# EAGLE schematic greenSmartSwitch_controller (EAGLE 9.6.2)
DATABASE: Z:\Eigene Dateien\Anwendungsdaten\Eagle\partdb\exp.txt
Assembly variants: Std

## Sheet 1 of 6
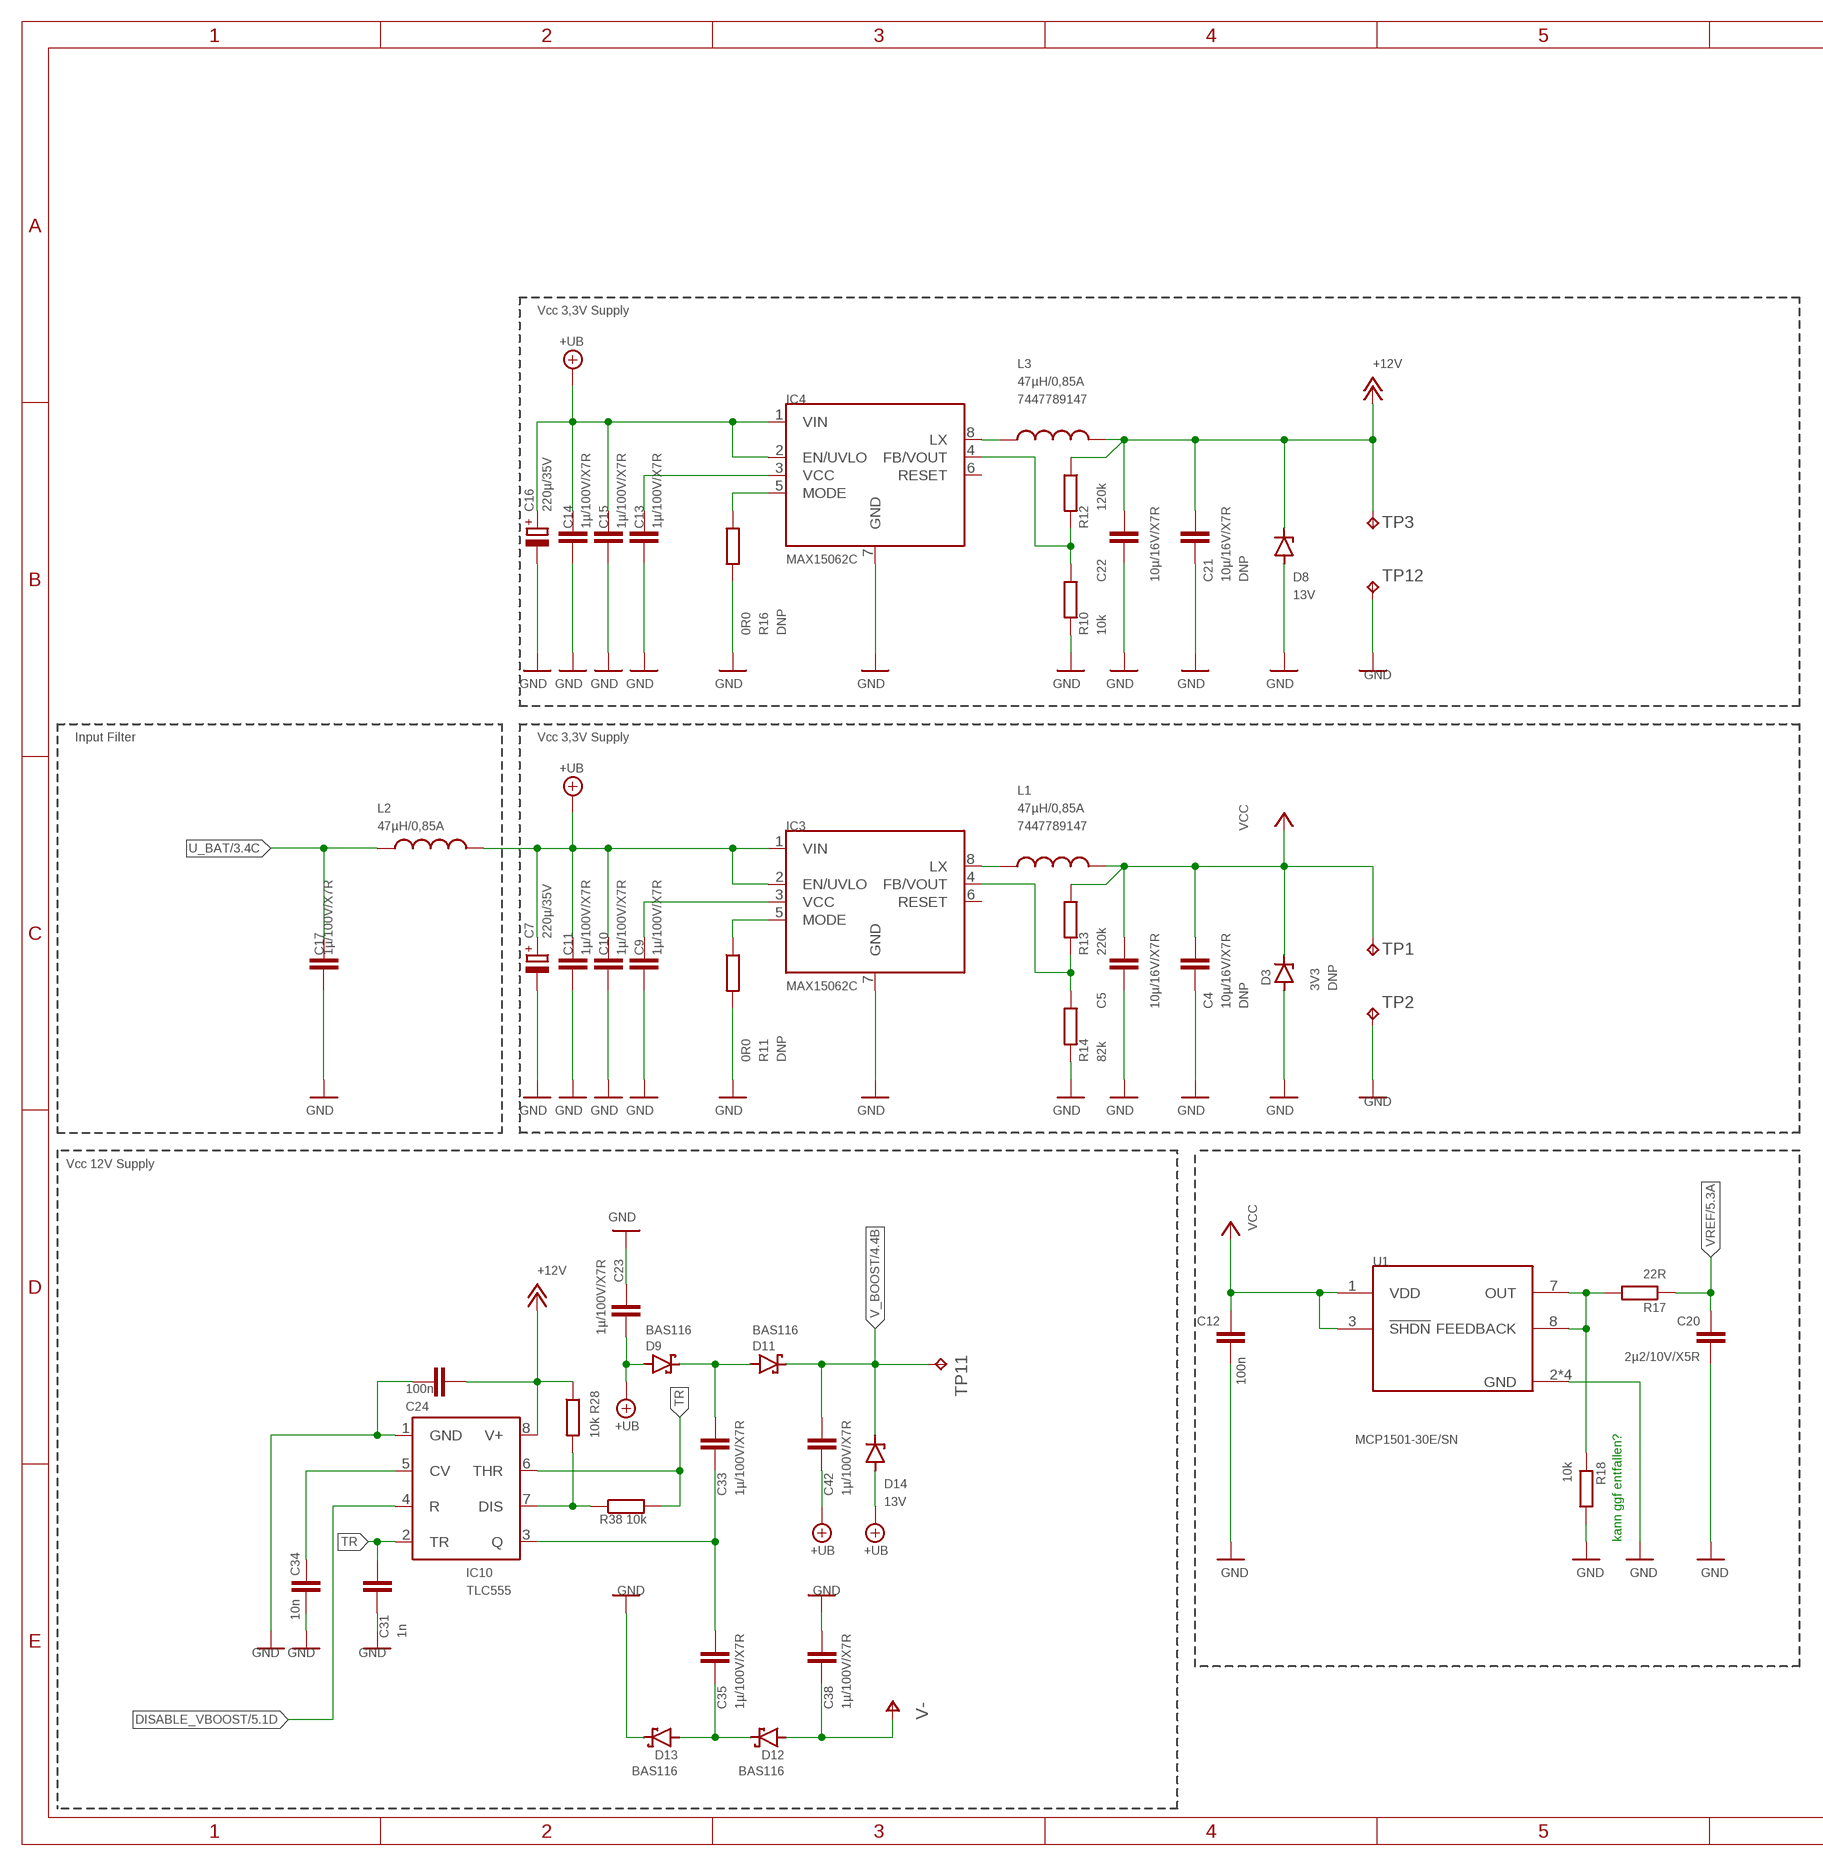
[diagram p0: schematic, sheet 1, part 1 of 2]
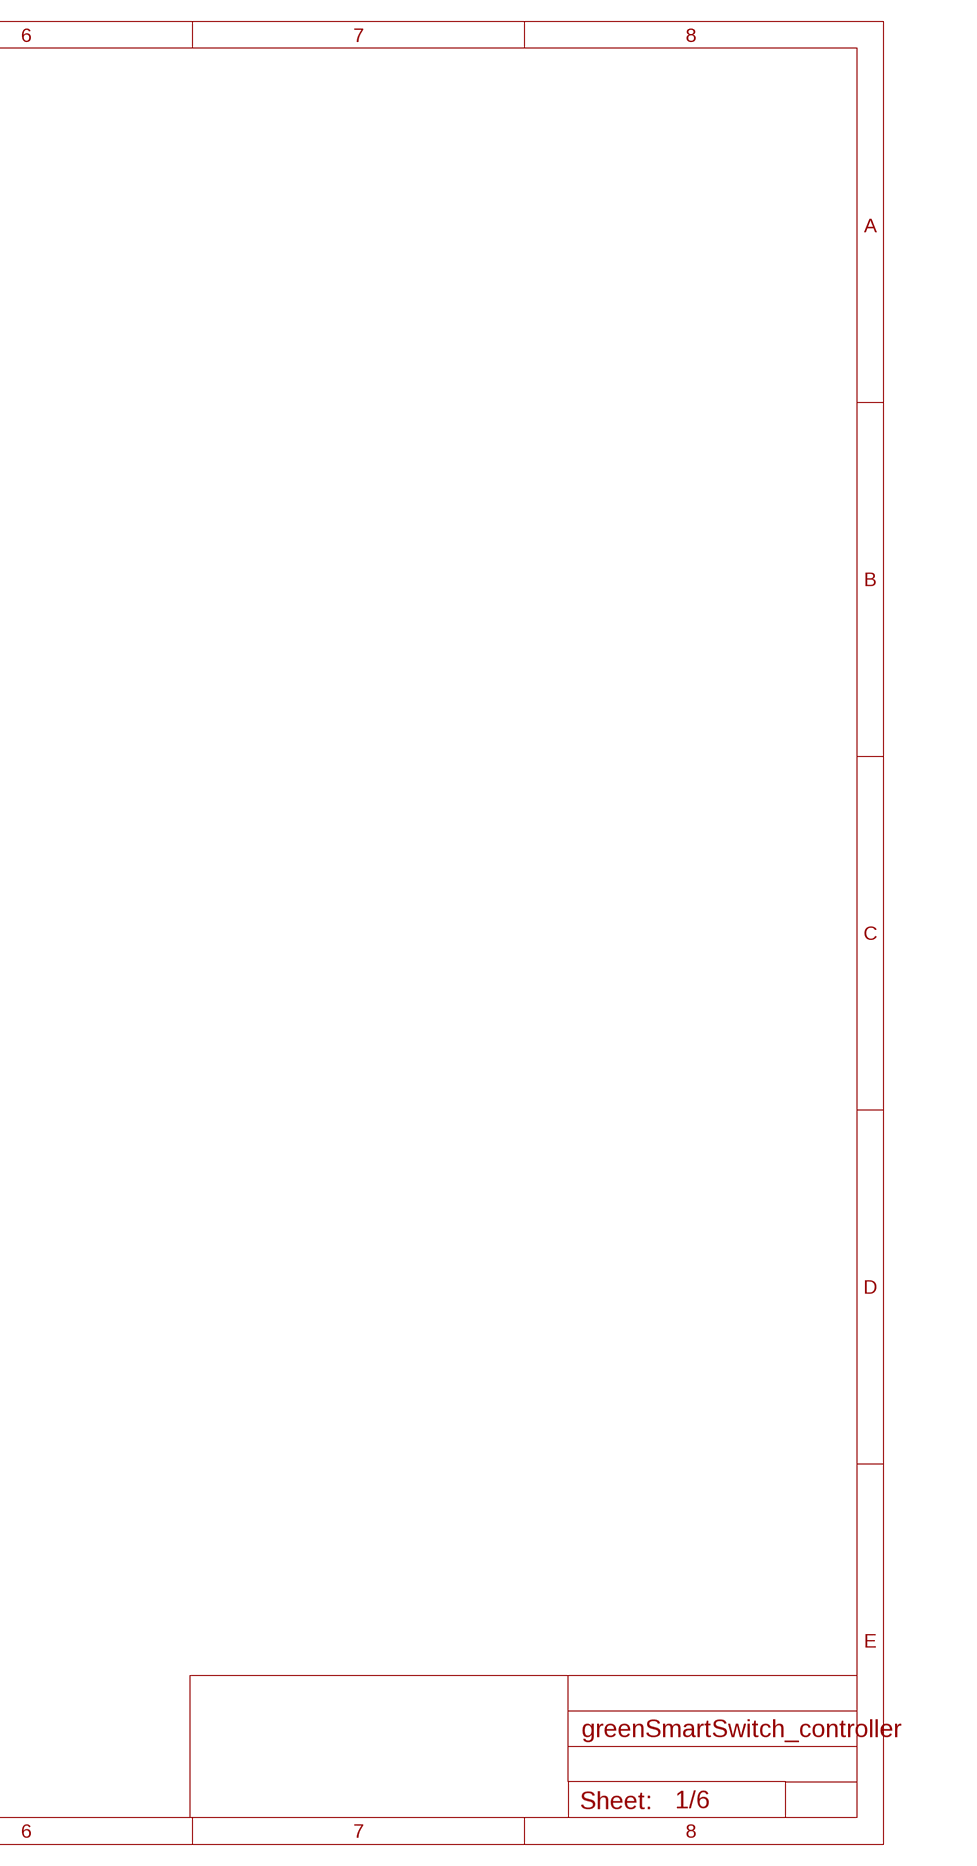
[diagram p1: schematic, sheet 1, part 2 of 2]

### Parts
C4  10µ/16V/X7R  C-EUC1210  [C1210]
C5  10µ/16V/X7R  C-EUC1210  [C1210]
C7  220µ/35V  CPOL-EUE3.5-8  [E3,5-8]
C9  1µ/100V/X7R  C-EUC1210  [C1210]
C10  1µ/100V/X7R  C-EUC1210  [C1210]
C11  1µ/100V/X7R  C-EUC1210  [C1210]
C12  100n  C-EUC0603  [C0603]
C13  1µ/100V/X7R  C-EUC1210  [C1210]
C14  1µ/100V/X7R  C-EUC1210  [C1210]
C15  1µ/100V/X7R  C-EUC1210  [C1210]
C16  220µ/35V  CPOL-EUE3.5-8  [E3,5-8]
C17  1µ/100V/X7R  C-EUC1210  [C1210]
C20  2µ2/10V/X5R  C-EUC0603  [C0603]
C21  10µ/16V/X7R  C-EUC1210  [C1210]
C22  10µ/16V/X7R  C-EUC1210  [C1210]
C23  1µ/100V/X7R  C-EUC1210  [C1210]
C24  100n  C-EUC0603  [C0603]
C31  1n  C-EUC0603  [C0603]
C33  1µ/100V/X7R  C-EUC1210  [C1210]
C34  10n  C-EUC0603  [C0603]
C35  1µ/100V/X7R  C-EUC1210  [C1210]
C38  1µ/100V/X7R  C-EUC1210  [C1210]
C42  1µ/100V/X7R  C-EUC1210  [C1210]
D3  3V3  ZENER-DIODESOD80C  [SOD80C]
D8  13V  ZENER-DIODESOD80C  [SOD80C]
D9  BAS116  BAS70  [SOT23]
D11  BAS116  BAS70  [SOT23]
D12  BAS116  BAS70  [SOT23]
D13  BAS116  BAS70  [SOT23]
D14  13V  ZENER-DIODESOD80C  [SOD80C]
IC3  MAX15062C  MAX15062A  [8TDFN]
IC4  MAX15062C  MAX15062A  [8TDFN]
IC10  TLC555  [SO8]
L1  47µH/0,85A  WE-PD_7332_PLASTIC_7447789147  [WE-PD_7332/7345_PLASTIC_BASE]
L2  47µH/0,85A  WE-PD_7332_PLASTIC_7447789147  [WE-PD_7332/7345_PLASTIC_BASE]
L3  47µH/0,85A  WE-PD_7332_PLASTIC_7447789147  [WE-PD_7332/7345_PLASTIC_BASE]
R10  10k  R-EU_R0603  [R0603]
R11  0R0  R-EU_R0603  [R0603]
R12  120k  R-EU_R0603  [R0603]
R13  220k  R-EU_R0603  [R0603]
R14  82k  R-EU_R0603  [R0603]
R16  0R0  R-EU_R0603  [R0603]
R17  22R  R-EU_R0603  [R0603]
R18  10k  R-EU_R0603  [R0603]
R28  10k  R-EU_R0603  [R0603]
R38  10k  R-EU_R0603  [R0603]
TP1  TP_0.6  [TP_0.6]
TP2  TP_0.6  [TP_0.6]
TP3  TP_0.6  [TP_0.6]
TP11  TP_0.6  [TP_0.6]
TP12  TP_0.6  [TP_0.6]
U1  MCP1501-30E/SN  MCP1501-40E/SN  [SOIC127P600X175-8N]

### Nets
+12V: C21.2 C22.2 C24.1 D8.C IC10.8(V+) L3.2 R12.1 R28.1 TP3.TP ; also sheet 2,4
+UB: C7.+ C10.2 C11.2 C14.2 C15.2 C16.+ C23.2 C42.1 D9.1(A) D14.A IC3.1(VIN) IC3.2(EN/UVLO) IC4.1(VIN) IC4.2(EN/UVLO) L2.2 ; also sheet 2
DISABLE_VBOOST: IC10.4(R) ; also sheet 5
GND: C4.1 C5.1 C7.- C9.1 C10.1 C11.1 C12.2 C13.1 C14.1 C15.1 C16.- C17.1 C20.2 C21.1 C22.1 C23.1 C24.2 C31.1 C34.1 C38.2 D3.A D8.A D13.3(C) IC3.7(GND) IC4.7(GND) IC10.1(GND) R10.2 R11.2 R14.2 R16.2 R18.2 TP2.TP TP12.TP U1.2(GND) U1.4(GND) U1.5(GND) U1.6(GND) ; also sheet 2,3,4,5,6
N$2: IC10.7(DIS) R28.2 R38.1
N$6: IC3.5(MODE) R11.1
N$8: C9.2 IC3.3(VCC)
N$21: IC3.4(FB/VOUT) R13.2 R14.1
N$23: C33.2 D9.3(C) D11.1(A)
N$26: C35.1 D12.3(C) D13.1(A)
N$36: C34.2 IC10.5(CV)
N$39: C33.1 C35.2 IC10.3(Q)
N$51: IC4.8(LX) L3.1
N$58: IC4.5(MODE) R16.1
N$60: C13.2 IC4.3(VCC)
N$61: IC4.4(FB/VOUT) R10.1 R12.2
N$91: IC3.8(LX) L1.1
N$119: R17.2 R18.1 U1.7(OUT) U1.8(FEEDBACK)
TR: C31.2 IC10.2(TR) IC10.6(THR) R38.2
U_BAT: C17.2 L2.1 ; also sheet 3
V-: C38.1 D12.1(A) ; also sheet 4
V_BOOST: C42.2 D11.3(C) D14.C TP11.TP ; also sheet 4
VCC: C4.2 C5.2 C12.1 D3.C L1.2 R13.1 TP1.TP U1.1(VDD) U1.3(!SHDN) ; also sheet 2,3,5,6
VREF: C20.1 R17.1 ; also sheet 5,6
Unconnected: IC3.6(RESET) IC4.6(RESET)

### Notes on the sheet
- Vcc 3,3V Supply
- 7447789147
- Input Filter | Vcc 3,3V Supply
- 7447789147
- Vcc 12V Supply
- kann ggf entfallen?

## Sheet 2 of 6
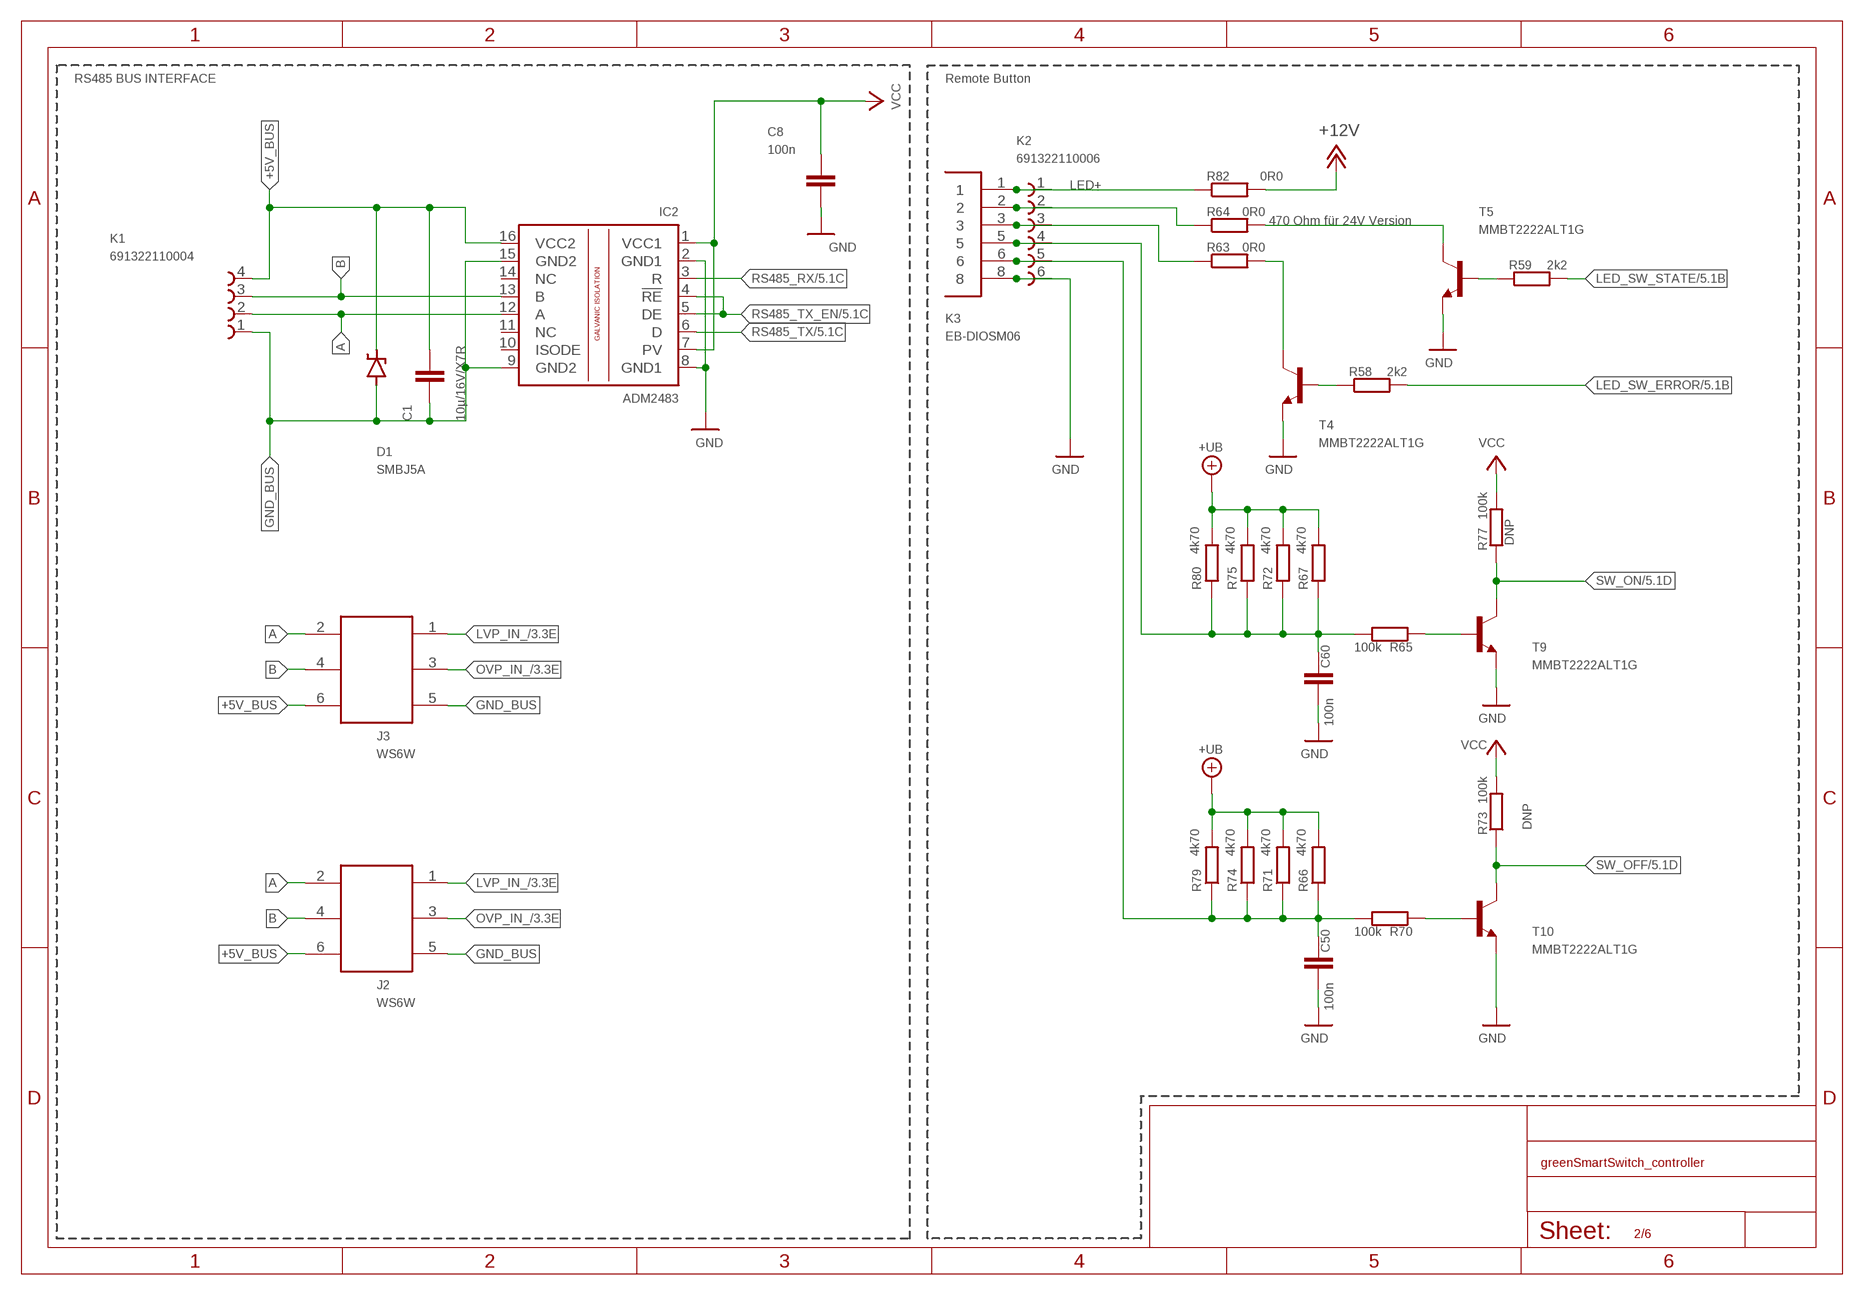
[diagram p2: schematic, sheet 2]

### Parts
C1  10µ/16V/X7R  C-EUC1210  [C1210]
C8  100n  C-EUC0603  [C0603]
C50  100n  C-EUC0603  [C0603]
C60  100n  C-EUC0603  [C0603]
D1  SMBJ5A  SUPPRESSOR-SMBJ  [SMBJ]
IC2  ADM2483  ISO1176  [SO-16DW]
J2  WS6W  61200621721  [61200621721]
J3  WS6W  61200621721  [61200621721]
K1  691322110004  [691322110004]
K2  691322110006  [691322110006]
K3  EB-DIOSM06  [PS/2-6]
R58  2k2  R-EU_R0603  [R0603]
R59  2k2  R-EU_R0603  [R0603]
R63  0R0  R-EU_R0603  [R0603]
R64  0R0  R-EU_R0603  [R0603]
R65  100k  R-EU_R0603  [R0603]
R66  4k70  R-EU_R1206  [R1206]
R67  4k70  R-EU_R1206  [R1206]
R70  100k  R-EU_R0603  [R0603]
R71  4k70  R-EU_R1206  [R1206]
R72  4k70  R-EU_R1206  [R1206]
R73  100k  R-EU_R0603  [R0603]
R74  4k70  R-EU_R1206  [R1206]
R75  4k70  R-EU_R1206  [R1206]
R77  100k  R-EU_R0603  [R0603]
R79  4k70  R-EU_R1206  [R1206]
R80  4k70  R-EU_R1206  [R1206]
R82  0R0  R-EU_R0603  [R0603]
T4  MMBT2222ALT1G  MMBT2222ALT1-NPN-SOT23-BEC  [SOT23-BEC]
T5  MMBT2222ALT1G  MMBT2222ALT1-NPN-SOT23-BEC  [SOT23-BEC]
T9  MMBT2222ALT1G  MMBT2222ALT1-NPN-SOT23-BEC  [SOT23-BEC]
T10  MMBT2222ALT1G  MMBT2222ALT1-NPN-SOT23-BEC  [SOT23-BEC]

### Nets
+5V_BUS: C1.2 D1.C IC2.16(VCC2) J2.6 J3.6 K1.4
+12V: R82.2 ; also sheet 1,4
+UB: R66.2 R67.2 R71.2 R72.2 R74.2 R75.2 R79.2 R80.2 ; also sheet 1
A: IC2.12(A) J2.2 J3.2 K1.2
B: IC2.13(B) J2.4 J3.4 K1.3
GND: C8.2 C50.2 C60.2 IC2.2(GND1) IC2.8(GND1) K2.6 K3.8 T4.E T5.E T9.E T10.E ; also sheet 1,3,4,5,6
GND_BUS: C1.1 D1.A IC2.9(GND2) IC2.15(GND2) J2.5 J3.5 K1.1
LED_SW_ERROR: R58.2 ; also sheet 5
LED_SW_STATE: R59.2 ; also sheet 5
LVP_IN_: J2.1 J3.1 ; also sheet 3
N$4: C60.1 K2.4 K3.5 R65.2 R67.1 R72.1 R75.1 R80.1
N$9: K2.1 K3.1 R82.1
N$14: C50.1 K2.5 K3.6 R66.1 R70.2 R71.1 R74.1 R79.1
N$15: R64.2 T5.C
N$17: K2.2 K3.2 R64.1
N$18: K2.3 K3.3 R63.1
N$25: R63.2 T4.C
N$27: R58.1 T4.B
N$30: R65.1 T9.B
N$32: R70.1 T10.B
N$33: R59.1 T5.B
OVP_IN_: J2.3 J3.3 ; also sheet 3
RS485_RX: IC2.3(R) ; also sheet 5
RS485_TX: IC2.6(D) ; also sheet 5
RS485_TX_EN: IC2.4(!RE) IC2.5(DE) ; also sheet 5
SW_OFF: R73.1 T10.C ; also sheet 5
SW_ON: R77.1 T9.C ; also sheet 5
VCC: C8.1 IC2.1(VCC1) IC2.7(PV) R73.2 R77.2 ; also sheet 1,3,5,6
Unconnected: IC2.10(ISODE) IC2.11(NC) IC2.14(NC)

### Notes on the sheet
- RS485 BUS INTERFACE | Remote Button
- LED+
- 470 Ohm für 24V Version

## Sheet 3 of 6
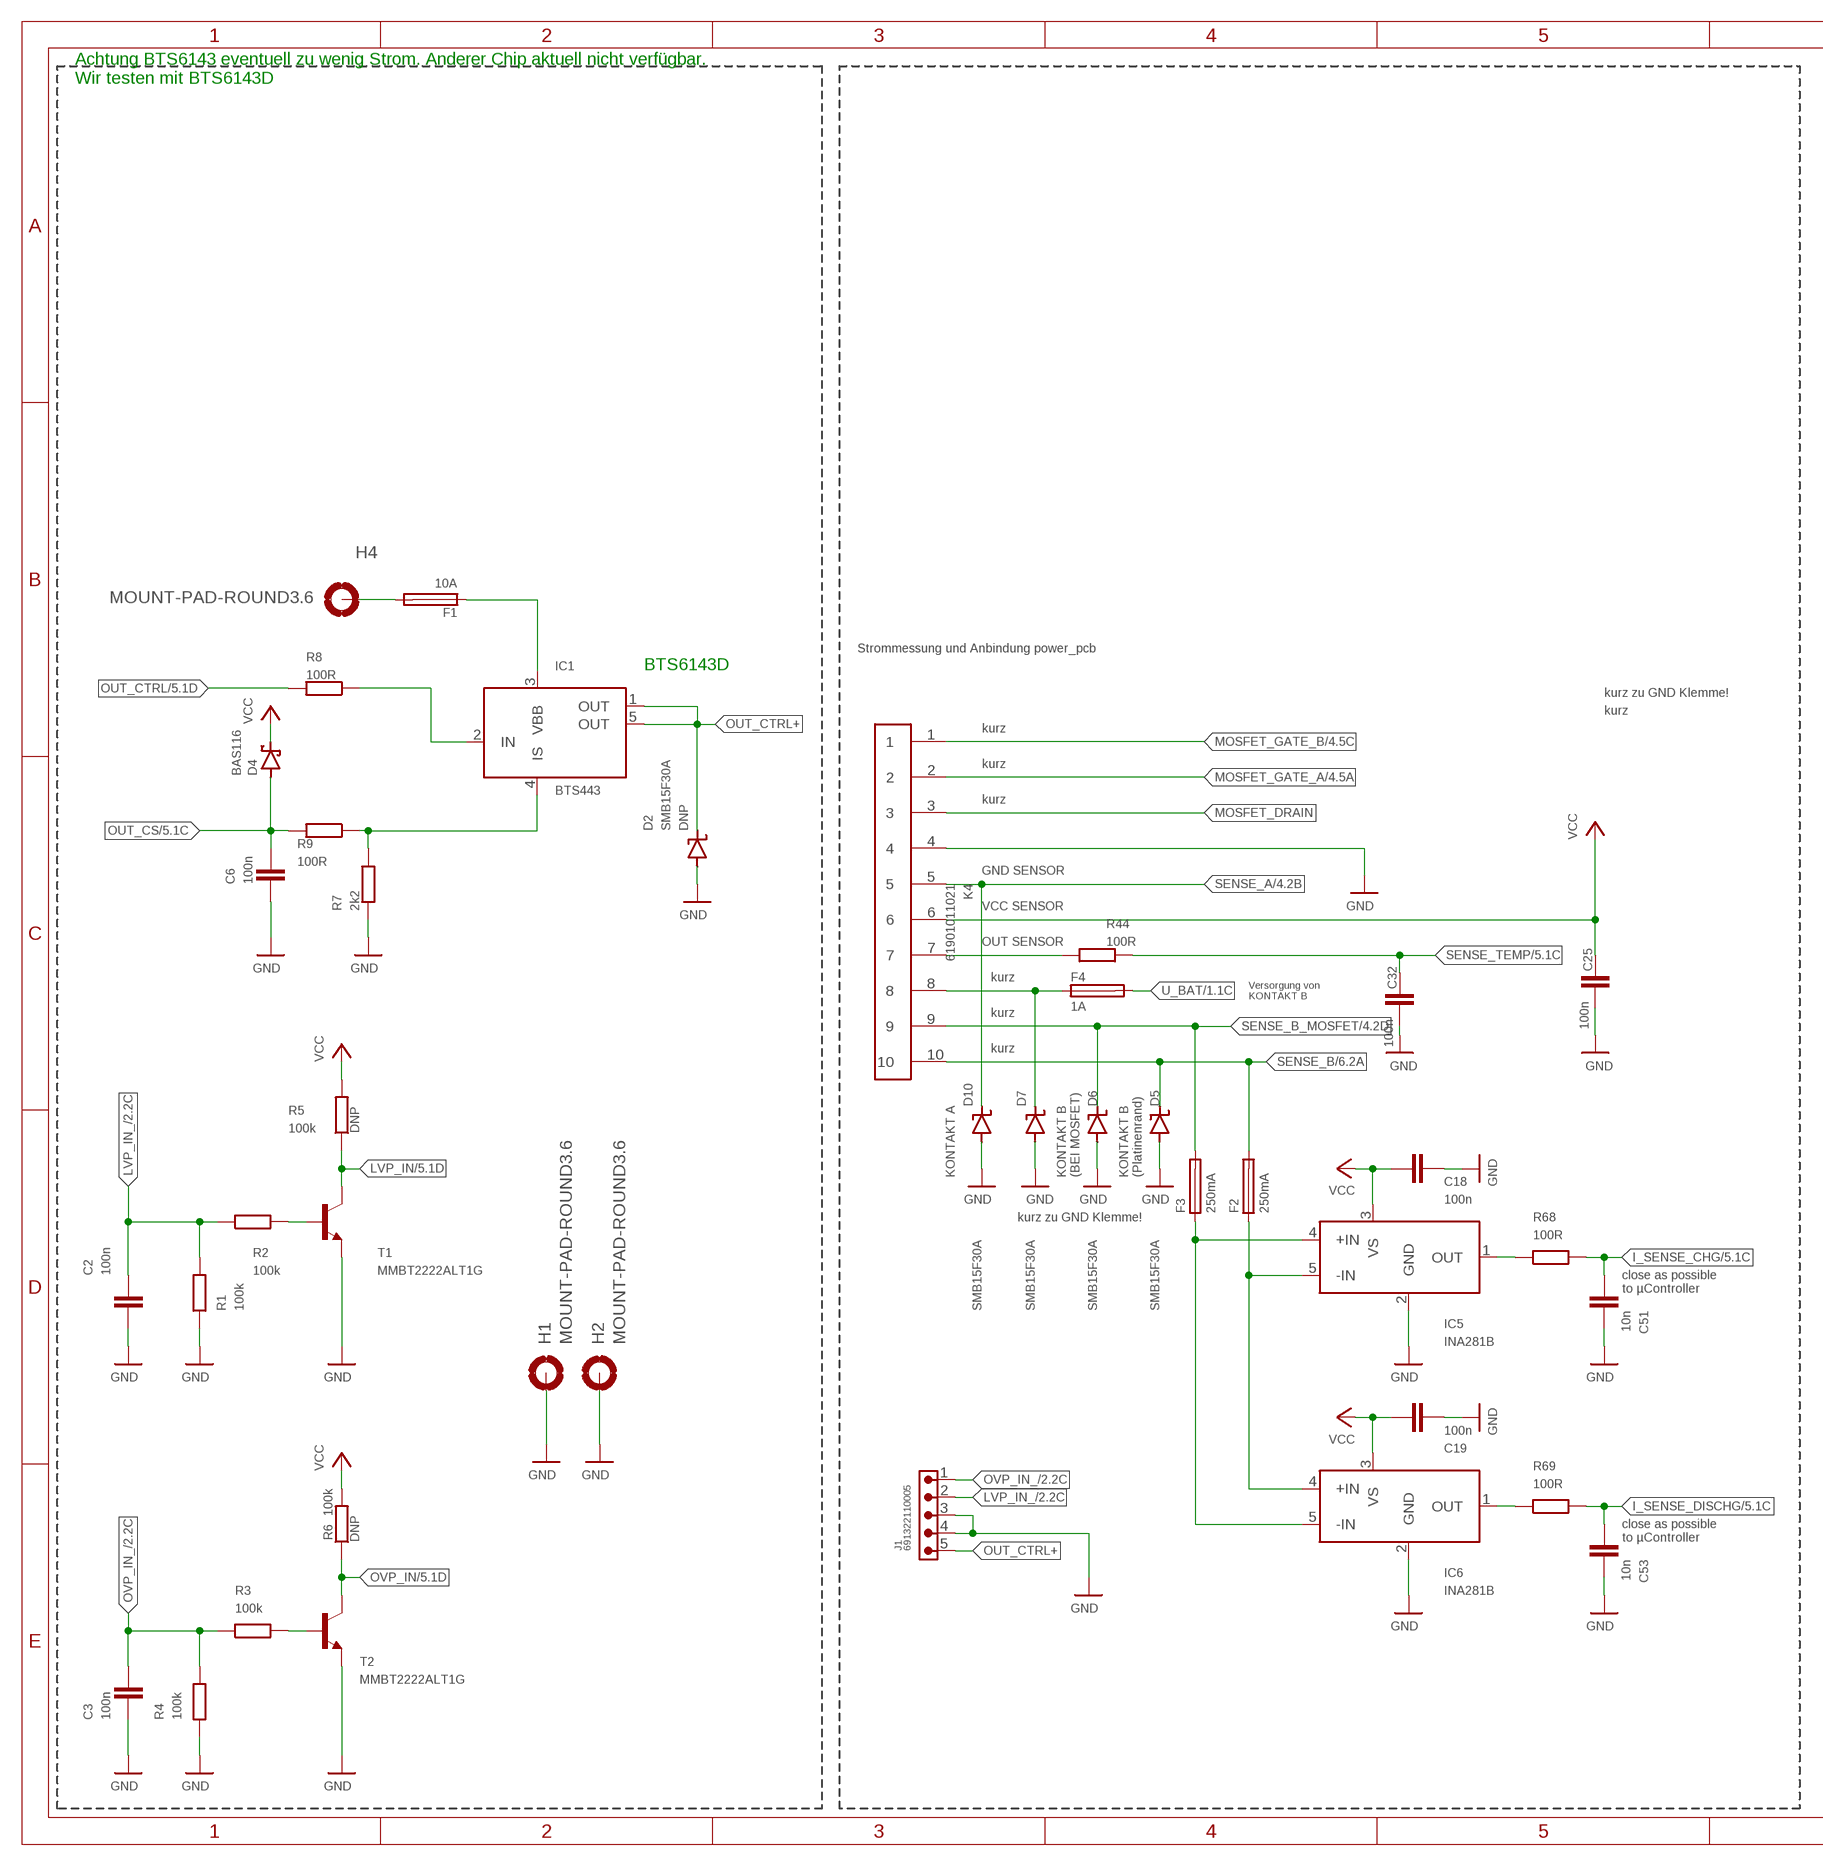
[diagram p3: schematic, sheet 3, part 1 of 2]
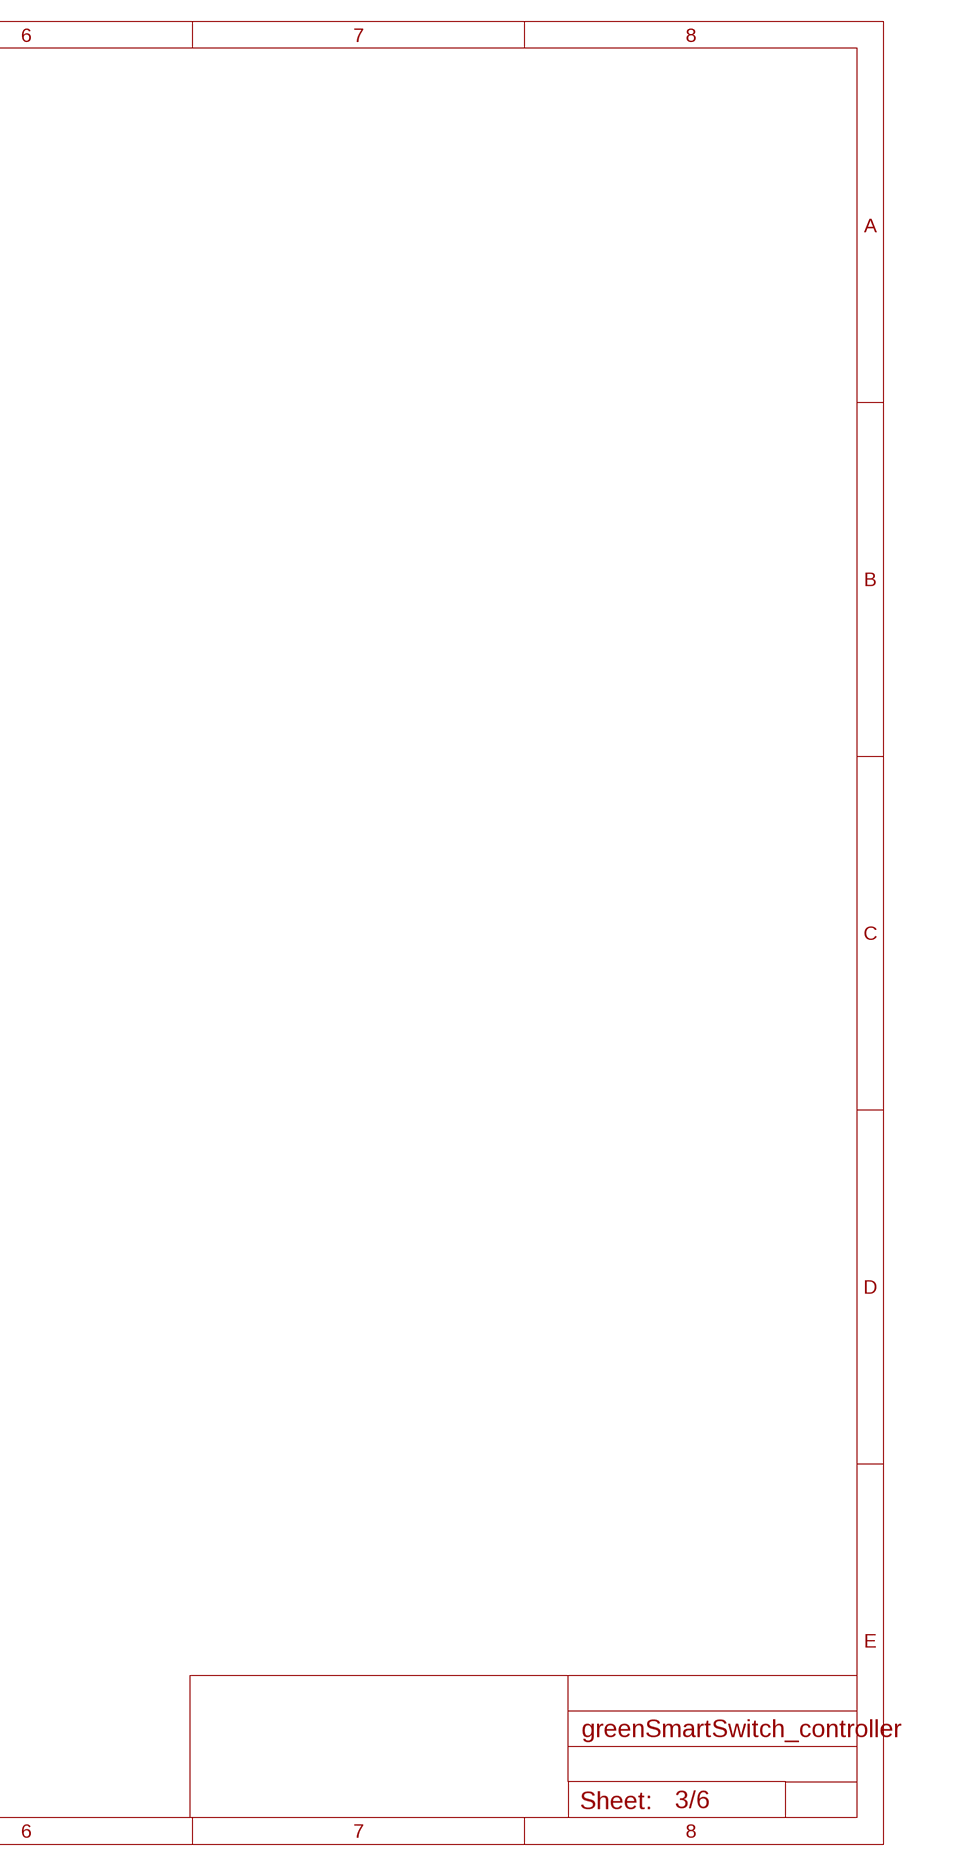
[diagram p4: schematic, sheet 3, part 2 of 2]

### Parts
C2  100n  C-EUC0603  [C0603]
C3  100n  C-EUC0603  [C0603]
C6  100n  C-EUC0603  [C0603]
C18  100n  C-EUC0603  [C0603]
C19  100n  C-EUC0603  [C0603]
C25  100n  C-EUC0603  [C0603]
C32  100n  C-EUC0603  [C0603]
C51  10n  C-EUC0603  [C0603]
C53  10n  C-EUC0603  [C0603]
D2  SMB15F30A  SUPPRESSOR-SMBJ  [SMBJ]
D4  BAS116  BAS70  [SOT23]
D5  SMB15F30A  SUPPRESSOR-SMBJ  [SMBJ]
D6  SMB15F30A  SUPPRESSOR-SMBJ  [SMBJ]
D7  SMB15F30A  SUPPRESSOR-SMBJ  [SMBJ]
D10  SMB15F30A  SUPPRESSOR-SMBJ  [SMBJ]
F1  10A  SSQ250-1K  [SSQ(2410)]
F2  250mA  SSQ250-1K  [SSQ(2410)]
F3  250mA  SSQ250-1K  [SSQ(2410)]
F4  1A  SSQ250-1K  [SSQ(2410)]
H1  MOUNT-PAD-ROUND3.6  [3,6-PAD]
H2  MOUNT-PAD-ROUND3.6  [3,6-PAD]
H4  MOUNT-PAD-ROUND3.6  [3,6-PAD]
IC1  BTS443  [PG-TO252-5-11]
IC5  INA281B  [SOT23-5]
IC6  INA281B  [SOT23-5]
J1  691322110005  [691322110005]
K4  61901011021  [61901011021]
R1  100k  R-EU_R0603  [R0603]
R2  100k  R-EU_R0603  [R0603]
R3  100k  R-EU_R0603  [R0603]
R4  100k  R-EU_R0603  [R0603]
R5  100k  R-EU_R0603  [R0603]
R6  100k  R-EU_R0603  [R0603]
R7  2k2  R-EU_R0603  [R0603]
R8  100R  R-EU_R0603  [R0603]
R9  100R  R-EU_R0603  [R0603]
R44  100R  R-EU_R0603  [R0603]
R68  100R  R-EU_R0603  [R0603]
R69  100R  R-EU_R0603  [R0603]
T1  MMBT2222ALT1G  MMBT2222ALT1-NPN-SOT23-BEC  [SOT23-BEC]
T2  MMBT2222ALT1G  MMBT2222ALT1-NPN-SOT23-BEC  [SOT23-BEC]

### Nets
GND: C2.1 C3.1 C6.1 C18.2 C19.2 C25.2 C32.2 C51.1 C53.1 D2.A D5.A D6.A D7.A D10.A H1.B3,6(MOUNT) H2.B3,6(MOUNT) IC5.2(GND) IC6.2(GND) J1.3 J1.4 K4.4 R1.1 R4.1 R7.2 T1.E T2.E ; also sheet 1,2,4,5,6
I_SENSE_CHG: C51.2 R68.2 ; also sheet 5
I_SENSE_DISCHG: C53.2 R69.2 ; also sheet 5
LVP_IN: R5.1 T1.C ; also sheet 5
LVP_IN_: C2.2 J1.2 R1.2 R2.1 ; also sheet 2
MOSFET_DRAIN: K4.3
MOSFET_GATE_A: K4.2 ; also sheet 4
MOSFET_GATE_B: K4.1 ; also sheet 4
N$1: K4.7 R44.2
N$10: IC6.1(OUT) R69.1
N$13: F3.1 IC5.4(+IN) IC6.5(-IN)
N$20: F1.2 H4.B3,6(MOUNT)
N$24: F2.1 IC5.5(-IN) IC6.4(+IN)
N$35: R2.2 T1.B
N$37: IC5.1(OUT) R68.1
N$40: R3.2 T2.B
N$47: D7.C F4.1 K4.8
N$68: IC1.4(IS) R7.1 R9.1
N$70: IC1.2(IN) R8.1
N$71: F1.1 IC1.3(VBB)
OUT_CS: C6.2 D4.1(A) R9.2 ; also sheet 5
OUT_CTRL: R8.2 ; also sheet 5
OUT_CTRL+: D2.C IC1.1(OUT) IC1.5(OUT) J1.5
OVP_IN: R6.1 T2.C ; also sheet 5
OVP_IN_: C3.2 J1.1 R3.1 R4.2 ; also sheet 2
SENSE_A: D10.C K4.5 ; also sheet 4,6
SENSE_B: D5.C F2.2 K4.10 ; also sheet 6
SENSE_B_MOSFET: D6.C F3.2 K4.9 ; also sheet 4
SENSE_TEMP: C32.1 R44.1 ; also sheet 5
U_BAT: F4.2 ; also sheet 1
VCC: C18.1 C19.1 C25.1 D4.3(C) IC5.3(VS) IC6.3(VS) K4.6 R5.2 R6.2 ; also sheet 1,2,5,6

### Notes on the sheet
- Achtung BTS6143 eventuell zu wenig Strom. Anderer Chip aktuell nicht verfügbar. 
  Wir testen mit BTS6143D
- Strommessung und Anbindung power_pcb
- BTS6143D
- kurz zu GND Klemme!
- kurz
- kurz
- kurz
- kurz
- GND SENSOR
- VCC SENSOR
- OUT SENSOR
- kurz
- Versorgung von
  KONTAKT B
- kurz
- kurz
- KONTAKT A
- KONTAKT B
  (BEI MOSFET)
- KONTAKT B 
  (Platinenrand)
- kurz zu GND Klemme!
- close as possible
  to µController
- close as possible
  to µController

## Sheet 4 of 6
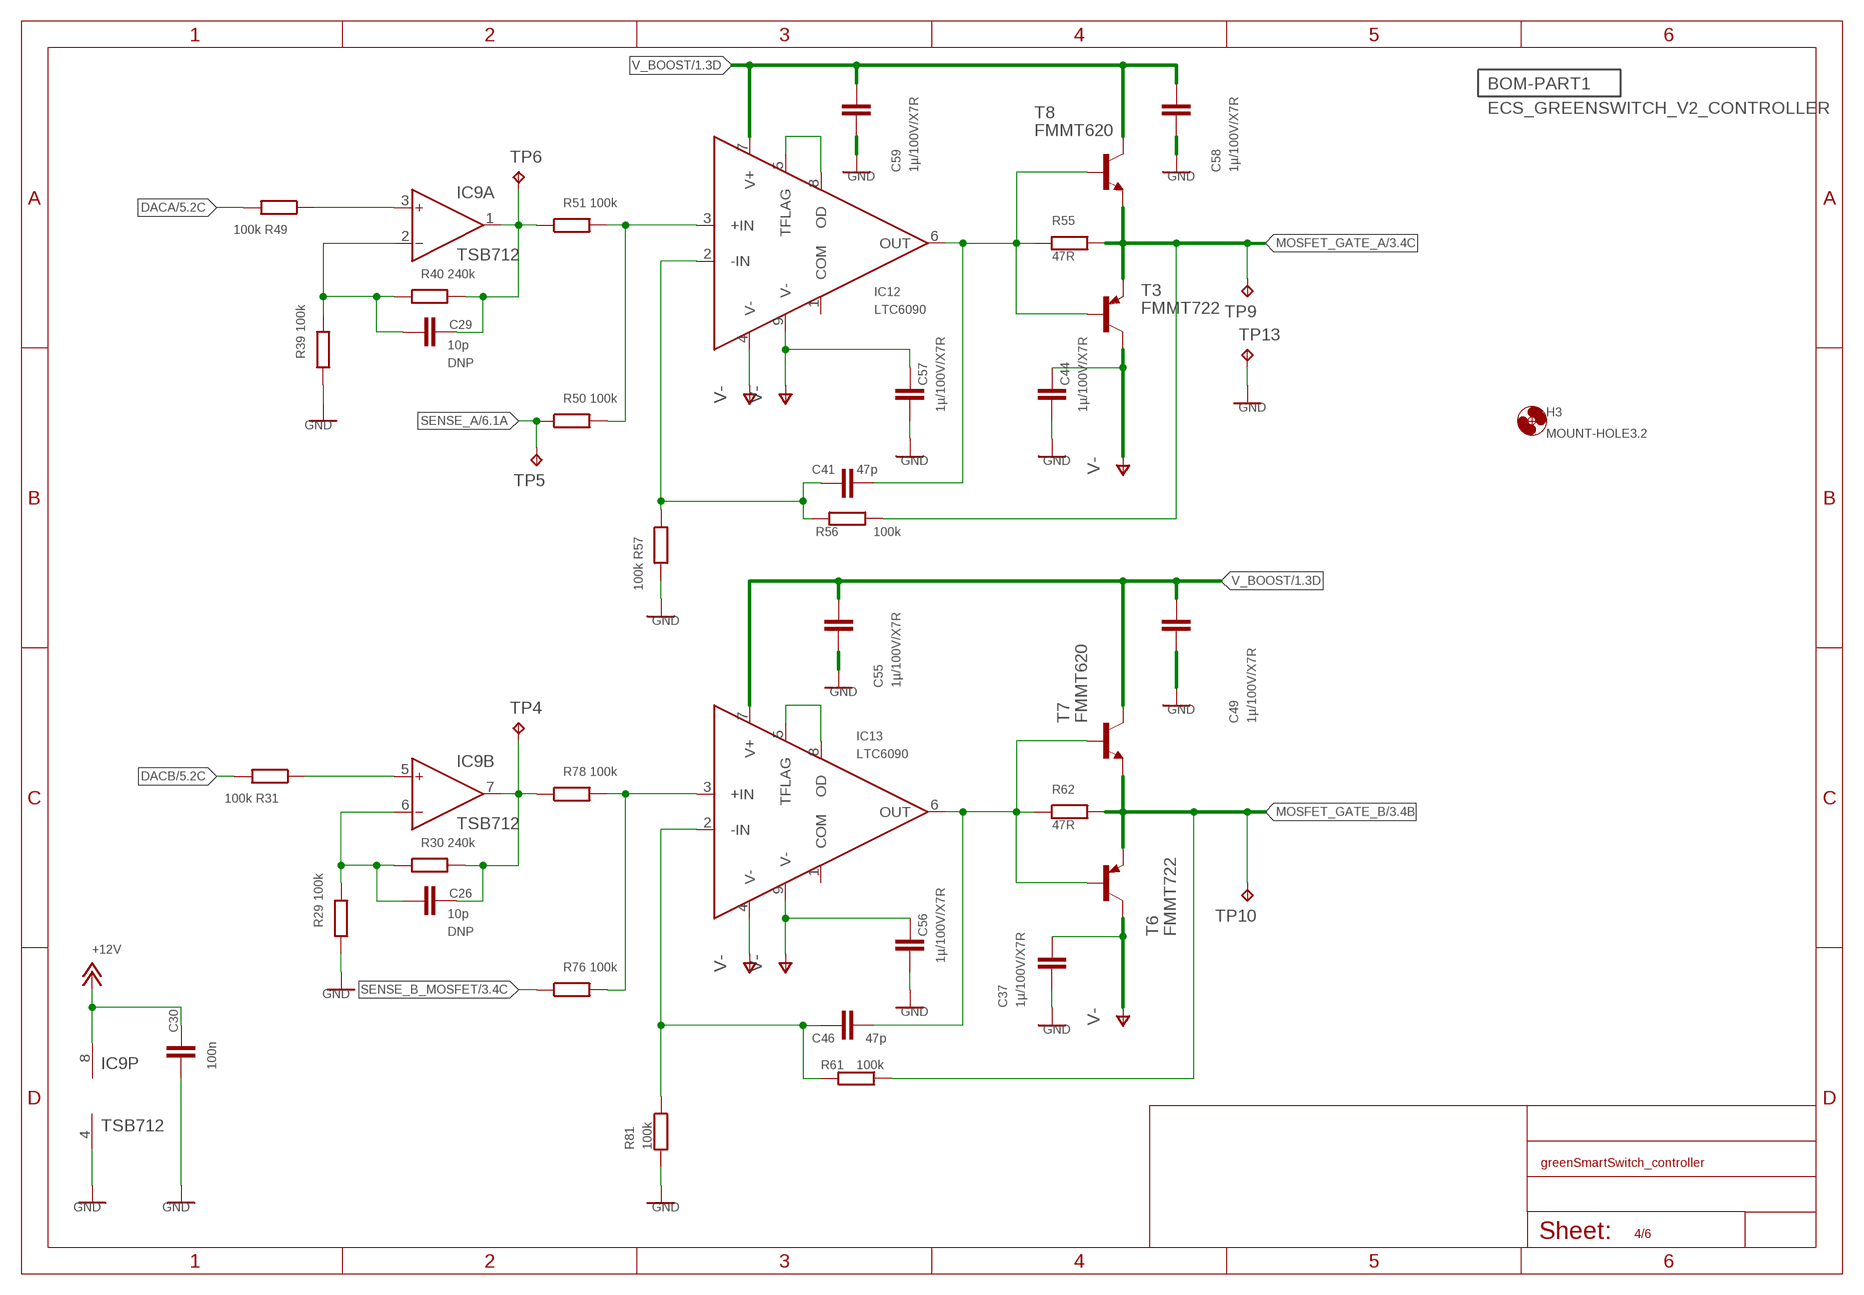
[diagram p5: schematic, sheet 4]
BOM-PART1 (BOM-PART): BOM: INCLUDE; PARTNO: PT066; QTY: 1

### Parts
C26  10p  C-EUC0603  [C0603]
C29  10p  C-EUC0603  [C0603]
C30  100n  C-EUC0603  [C0603]
C37  1µ/100V/X7R  C-EUC1210  [C1210]
C41  47p  C-EUC0603  [C0603]
C44  1µ/100V/X7R  C-EUC1210  [C1210]
C46  47p  C-EUC0603  [C0603]
C49  1µ/100V/X7R  C-EUC1210  [C1210]
C55  1µ/100V/X7R  C-EUC1210  [C1210]
C56  1µ/100V/X7R  C-EUC1210  [C1210]
C57  1µ/100V/X7R  C-EUC1210  [C1210]
C58  1µ/100V/X7R  C-EUC1210  [C1210]
C59  1µ/100V/X7R  C-EUC1210  [C1210]
H3  MOUNT-HOLE3.2  [3,2]
IC9  TSB712  TS912  [SO8]
IC12  LTC6090  [S8E(SOIC)]
IC13  LTC6090  [S8E(SOIC)]
R29  100k  R-EU_R0603  [R0603]
R30  240k  R-EU_R0603  [R0603]
R31  100k  R-EU_R0603  [R0603]
R39  100k  R-EU_R0603  [R0603]
R40  240k  R-EU_R0603  [R0603]
R49  100k  R-EU_R0603  [R0603]
R50  100k  R-EU_R0603  [R0603]
R51  100k  R-EU_R0603  [R0603]
R55  47R  R-EU_R0603  [R0603]
R56  100k  R-EU_R0603  [R0603]
R57  100k  R-EU_R0603  [R0603]
R61  100k  R-EU_R0603  [R0603]
R62  47R  R-EU_R0603  [R0603]
R76  100k  R-EU_R0603  [R0603]
R78  100k  R-EU_R0603  [R0603]
R81  100k  R-EU_R0603  [R0603]
T3  FMMT722  BC857A-PNP-SOT23-BEC  [SOT23-BEC]
T6  FMMT722  BC857A-PNP-SOT23-BEC  [SOT23-BEC]
T7  FMMT620  BC847  [SOT23]
T8  FMMT620  BC847  [SOT23]
TP4  TP_0.6  [TP_0.6]
TP5  TP_0.6  [TP_0.6]
TP6  TP_0.6  [TP_0.6]
TP9  TP_0.6  [TP_0.6]
TP10  TP_0.6  [TP_0.6]
TP13  TP_0.6  [TP_0.6]

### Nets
+12V: C30.1 IC9.8(P:V+) ; also sheet 1,2
DACA: R49.2 ; also sheet 5
DACA_: IC9.3(A:IN+) R49.1
DACB: R31.2 ; also sheet 5
DACB_: IC9.5(B:IN+) R31.1
GND: C30.2 C37.2 C44.2 C49.2 C55.2 C56.2 C57.2 C58.2 C59.2 IC9.4(P:V-) R29.1 R39.1 R57.2 R81.2 TP13.TP ; also sheet 1,2,3,5,6
MOSFET_GATE_A: R55.2 R56.1 T3.E T8.2(E) TP9.TP ; also sheet 3
MOSFET_GATE_B: R61.1 R62.2 T6.E T7.2(E) TP10.TP ; also sheet 3
N$19: C46.2 IC13.2(-IN) R61.2 R81.1
N$22: C41.2 IC12.2(-IN) R56.2 R57.1
N$29: C29.1 IC9.1(A:OUT) R40.2 R51.1 TP6.TP
N$38: IC12.5(TFLAG) IC12.8(OD)
N$43: C26.2 IC9.6(B:IN-) R29.2 R30.1
N$46: IC13.5(TFLAG) IC13.8(OD)
N$54: IC12.3(+IN) R50.2 R51.2
N$56: C26.1 IC9.7(B:OUT) R30.2 R78.1 TP4.TP
N$59: IC13.3(+IN) R76.2 R78.2
N$66: C29.2 IC9.2(A:IN-) R39.2 R40.1
PREDRIVER_A: C41.1 IC12.6(OUT) R55.1 T3.B T8.1(B)
PREDRIVER_B: C46.1 IC13.6(OUT) R62.1 T6.B T7.1(B)
SENSE_A: R50.1 TP5.TP ; also sheet 3,6
SENSE_B_MOSFET: R76.1 ; also sheet 3
V-: C37.1 C44.1 C56.1 C57.1 IC12.4(V-) IC12.9(V-) IC13.4(V-) IC13.9(V-) T3.C T6.C ; also sheet 1
V_BOOST: C49.1 C55.1 C58.1 C59.1 IC12.7(V+) IC13.7(V+) T7.3(C) T8.3(C) ; also sheet 1
Unconnected: IC12.1(COM) IC13.1(COM)

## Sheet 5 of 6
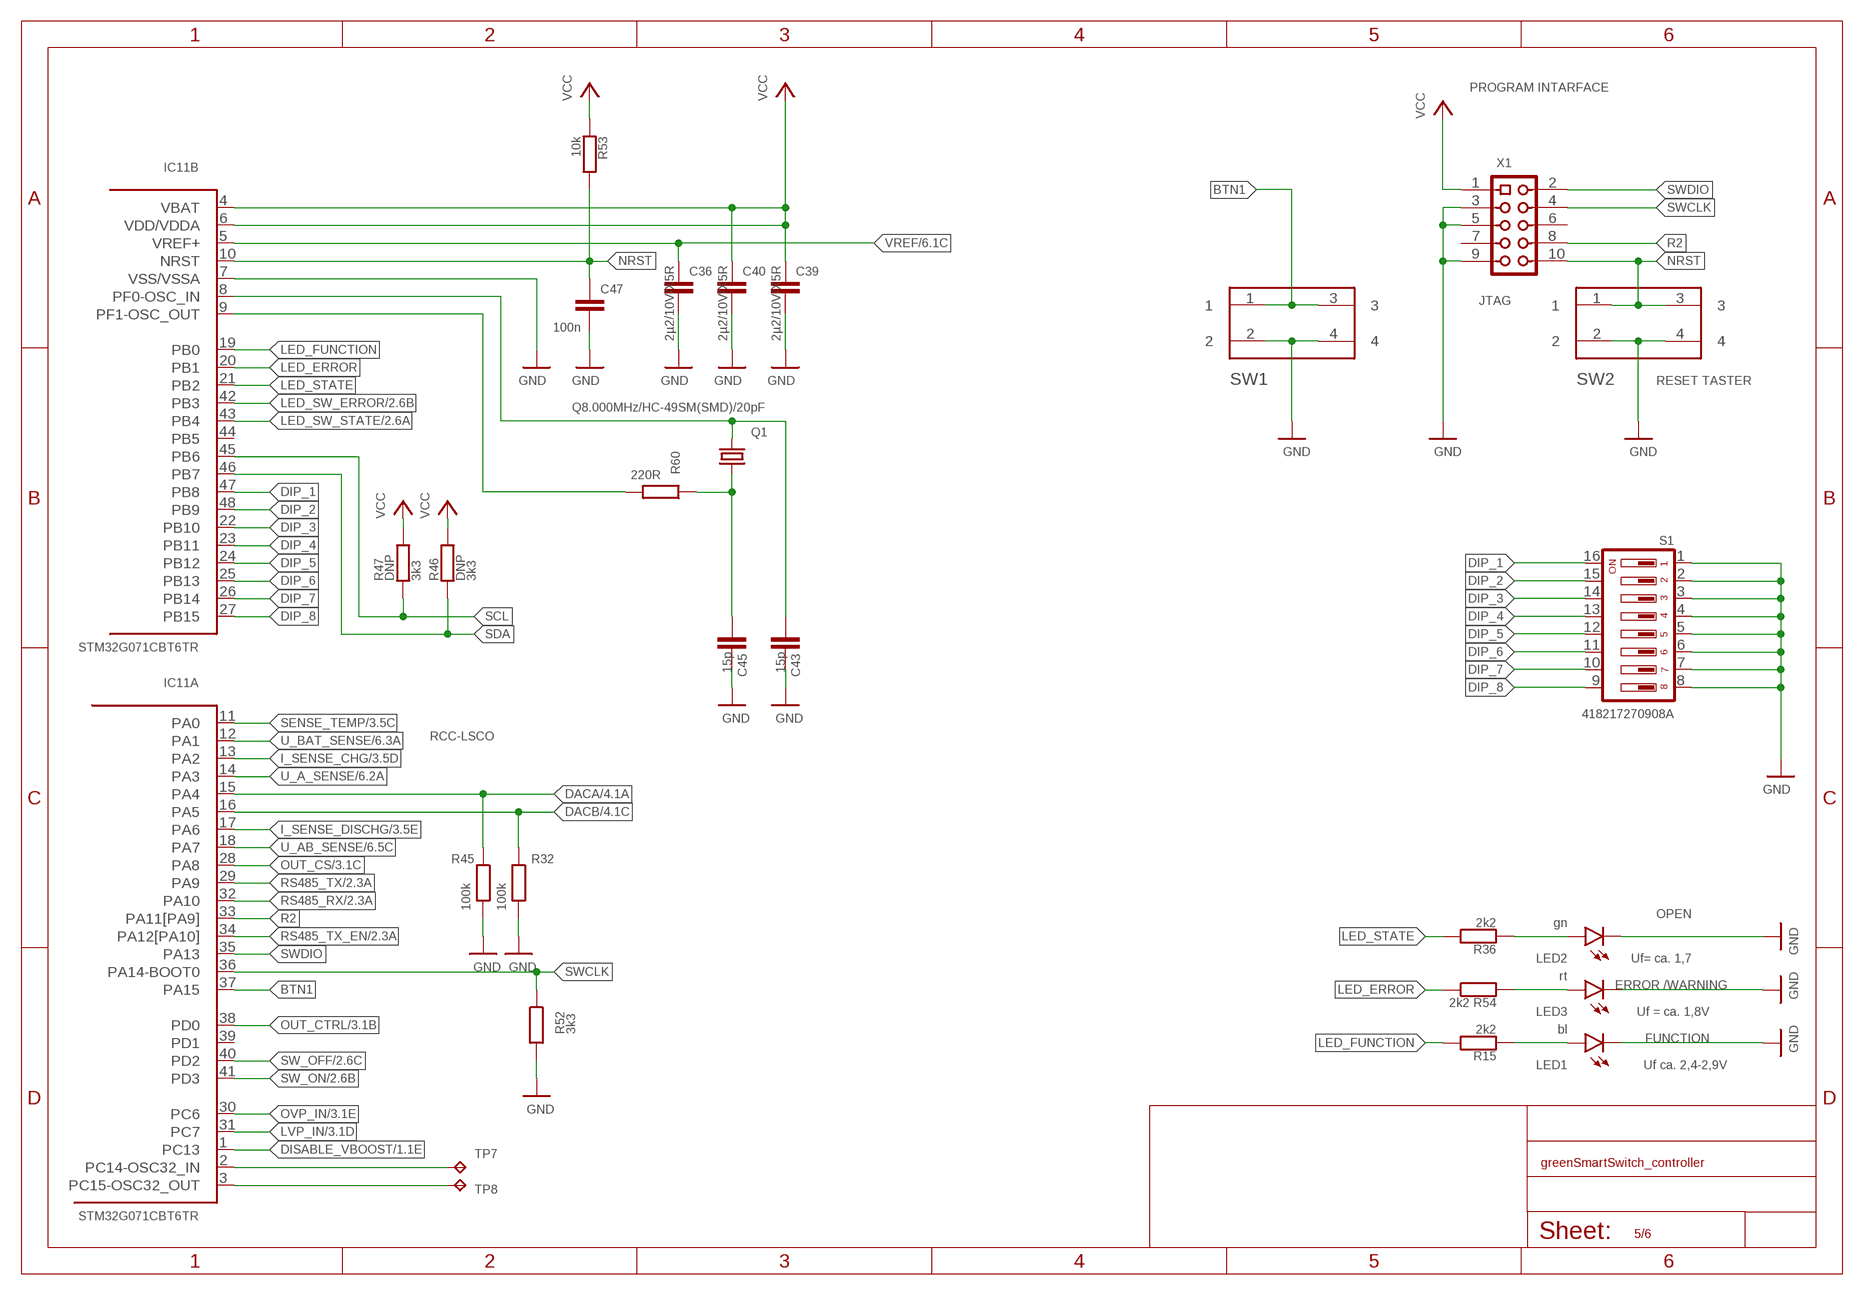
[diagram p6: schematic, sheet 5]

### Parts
C36  2µ2/10V/X5R  C-EUC0603  [C0603]
C39  2µ2/10V/X5R  C-EUC0603  [C0603]
C40  2µ2/10V/X5R  C-EUC0603  [C0603]
C43  15p  C-EUC0603  [C0603]
C45  15p  C-EUC0603  [C0603]
C47  100n  C-EUC0603  [C0603]
IC11  STM32G071CBT6TR  STM32G070CB  [LQFP48]
LED1  bl  LEDCHIPLED_0603  [CHIPLED_0603]
LED2  gn  LEDCHIPLED_0603  [CHIPLED_0603]
LED3  rt  LEDCHIPLED_0603  [CHIPLED_0603]
Q1  Q8.000MHz/HC-49SM(SMD)/20pF  CRYSTALHC49UP  [HC49UP]
R15  2k2  R-EU_R0603  [R0603]
R32  100k  R-EU_R0603  [R0603]
R36  2k2  R-EU_R0603  [R0603]
R45  100k  R-EU_R0603  [R0603]
R46  3k3  R-EU_R0603  [R0603]
R47  3k3  R-EU_R0603  [R0603]
R52  3k3  R-EU_R0603  [R0603]
R53  10k  R-EU_R0603  [R0603]
R54  2k2  R-EU_R0603  [R0603]
R60  220R  R-EU_R0603  [R0603]
S1  418217270908A  DA08  [DA-08]
SW1  430182095816  [430182095816]
SW2  430182095816  [430182095816]
TP7  TP_0.6  [TP_0.6]
TP8  TP_0.6  [TP_0.6]
X1  JTAG  PF2X5SMD1.27MM  [PF2X5SMD50MIL]

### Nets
BTN1: IC11.37(A:PA15) SW1.1 SW1.3
DACA: IC11.15(A:PA4) R45.1 ; also sheet 4
DACB: IC11.16(A:PA5) R32.1 ; also sheet 4
DIP_1: IC11.47(B:PB8) S1.16
DIP_2: IC11.48(B:PB9) S1.15
DIP_3: IC11.22(B:PB10) S1.14
DIP_4: IC11.23(B:PB11) S1.13
DIP_5: IC11.24(B:PB12) S1.12
DIP_6: IC11.25(B:PB13) S1.11
DIP_7: IC11.26(B:PB14) S1.10
DIP_8: IC11.27(B:PB15) S1.9
DISABLE_VBOOST: IC11.1(A:PC13) ; also sheet 1
GND: C36.2 C39.2 C40.2 C43.1 C45.1 C47.2 IC11.7(B:VSS/VSSA) LED1.C LED2.C LED3.C R32.2 R45.2 R52.2 S1.1 S1.2 S1.3 S1.4 S1.5 S1.6 S1.7 S1.8 SW1.2 SW1.4 SW2.2 SW2.4 X1.3 X1.5 X1.9 ; also sheet 1,2,3,4,6
I_SENSE_CHG: IC11.13(A:PA2) ; also sheet 3
I_SENSE_DISCHG: IC11.17(A:PA6) ; also sheet 3
LED_ERROR: IC11.20(B:PB1) R54.1
LED_FUNCTION: IC11.19(B:PB0) R15.1
LED_STATE: IC11.21(B:PB2) R36.1
LED_SW_ERROR: IC11.42(B:PB3) ; also sheet 2
LED_SW_STATE: IC11.43(B:PB4) ; also sheet 2
LVP_IN: IC11.31(A:PC7) ; also sheet 3
N$5: C43.2 IC11.8(B:PF0-OSC_IN) Q1.2
N$7: C45.2 Q1.1 R60.1
N$11: IC11.9(B:PF1-OSC_OUT) R60.2
N$12: LED2.A R36.2
N$16: IC11.2(A:PC14-OSC32_IN) TP7.TP
N$31: LED1.A R15.2
N$34: LED3.A R54.2
N$42: IC11.3(A:PC15-OSC32_OUT) TP8.TP
NRST: C47.1 IC11.10(B:NRST) R53.1 SW2.1 SW2.3 X1.10
OUT_CS: IC11.28(A:PA8) ; also sheet 3
OUT_CTRL: IC11.38(A:PD0) ; also sheet 3
OVP_IN: IC11.30(A:PC6) ; also sheet 3
R2: IC11.33(A:PA11[PA9]) X1.8
RS485_RX: IC11.32(A:PA10) ; also sheet 2
RS485_TX: IC11.29(A:PA9) ; also sheet 2
RS485_TX_EN: IC11.34(A:PA12[PA10]) ; also sheet 2
SCL: IC11.45(B:PB6) R47.1
SDA: IC11.46(B:PB7) R46.1
SENSE_TEMP: IC11.11(A:PA0) ; also sheet 3
SW_OFF: IC11.40(A:PD2) ; also sheet 2
SW_ON: IC11.41(A:PD3) ; also sheet 2
SWCLK: IC11.36(A:PA14-BOOT0) R52.1 X1.4
SWDIO: IC11.35(A:PA13) X1.2
U_A_SENSE: IC11.14(A:PA3) ; also sheet 6
U_AB_SENSE: IC11.18(A:PA7) ; also sheet 6
U_BAT_SENSE: IC11.12(A:PA1) ; also sheet 6
VCC: C39.1 C40.1 IC11.4(B:VBAT) IC11.6(B:VDD/VDDA) R46.2 R47.2 R53.2 X1.1 ; also sheet 1,2,3,6
VREF: C36.1 IC11.5(B:VREF+) ; also sheet 1,6
Unconnected: IC11.39(A:PD1) IC11.44(B:PB5) X1.6 X1.7

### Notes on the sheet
- PROGRAM INTARFACE
- RESET TASTER
- RCC-LSCO
- OPEN
- Uf= ca. 1,7
- ERROR /WARNING
- Uf = ca. 1,8V
- FUNCTION
- Uf ca. 2,4-2,9V

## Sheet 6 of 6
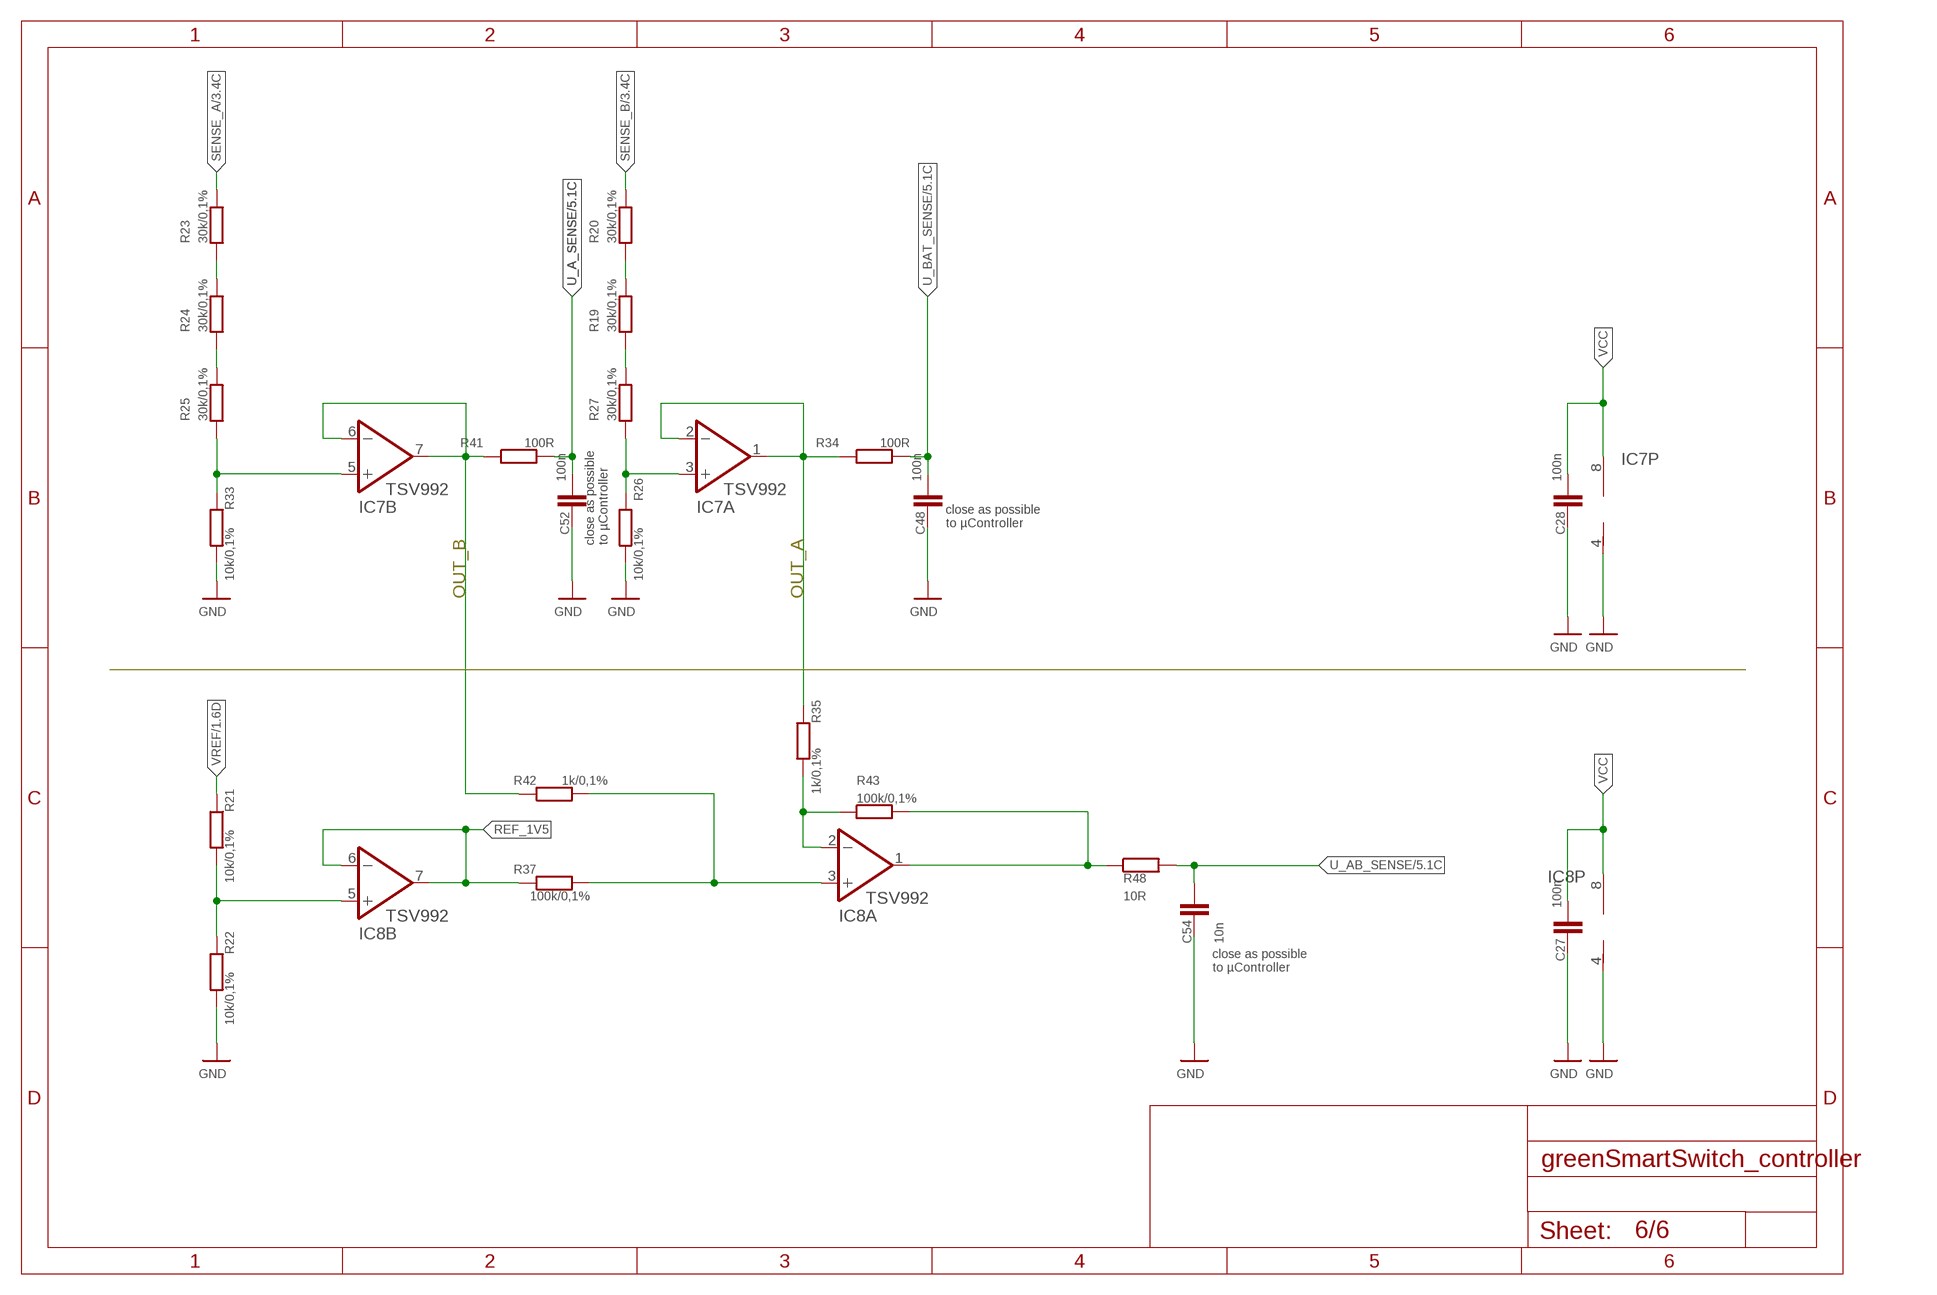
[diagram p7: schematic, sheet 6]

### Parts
C27  100n  C-EUC0603  [C0603]
C28  100n  C-EUC0603  [C0603]
C48  100n  C-EUC0603  [C0603]
C52  100n  C-EUC0603  [C0603]
C54  10n  C-EUC0603  [C0603]
IC7  TSV992  LT6231IS8  [S8]
IC8  TSV992  LT6231IS8  [S8]
R19  30k/0,1%  R-EU_R0603  [R0603]
R20  30k/0,1%  R-EU_R0603  [R0603]
R21  10k/0,1%  R-EU_R0603  [R0603]
R22  10k/0,1%  R-EU_R0603  [R0603]
R23  30k/0,1%  R-EU_R0603  [R0603]
R24  30k/0,1%  R-EU_R0603  [R0603]
R25  30k/0,1%  R-EU_R0603  [R0603]
R26  10k/0,1%  R-EU_R0603  [R0603]
R27  30k/0,1%  R-EU_R0603  [R0603]
R33  10k/0,1%  R-EU_R0603  [R0603]
R34  100R  R-EU_R0603  [R0603]
R35  1k/0,1%  R-EU_R0603  [R0603]
R37  100k/0,1%  R-EU_R0603  [R0603]
R41  100R  R-EU_R0603  [R0603]
R42  1k/0,1%  R-EU_R0603  [R0603]
R43  100k/0,1%  R-EU_R0603  [R0603]
R48  10R  R-EU_R0603  [R0603]

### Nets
GND: C27.1 C28.1 C48.1 C52.1 C54.1 IC7.4(P:V-) IC8.4(P:V-) R22.2 R26.2 R33.2 ; also sheet 1,2,3,4,5
N$3: R24.1 R25.2
N$28: IC7.1(A:OUT) IC7.2(A:-IN) R34.1 R35.1
N$41: IC7.6(B:-IN) IC7.7(B:OUT) R41.1 R42.1
N$44: IC8.2(A:-IN) R35.2 R43.1
N$45: IC8.3(A:+IN) R37.2 R42.2
N$48: IC7.3(A:+IN) R26.1 R27.1
N$49: R23.1 R24.2
N$50: R19.1 R27.2
N$52: R19.2 R20.1
N$55: IC8.5(B:+IN) R21.2 R22.1
N$57: IC7.5(B:+IN) R25.1 R33.1
N$9999: IC8.1(A:OUT) R43.2 R48.1
REF_1V5: IC8.6(B:-IN) IC8.7(B:OUT) R37.1
SENSE_A: R23.2 ; also sheet 3,4
SENSE_B: R20.2 ; also sheet 3
U_A_SENSE: C52.2 R41.2 ; also sheet 5
U_AB_SENSE: C54.2 R48.2 ; also sheet 5
U_BAT_SENSE: C48.2 R34.2 ; also sheet 5
VCC: C27.2 C28.2 IC7.8(P:V+) IC8.8(P:V+) ; also sheet 1,2,3,5
VREF: R21.1 ; also sheet 1,5

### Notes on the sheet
- close as possible
  to µController
- close as possible
  to µController
- OUT_B | OUT_A
- close as possible
  to µController

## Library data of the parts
C1 C5 C22 = rcl:C-EU: CAPACITOR, European symbol; PARTNO: C218; SPICEPREFIX: C
C2 C3 C6 C8 C25 C27 C28 C32 C48 C50 C52 C60 = resistor:C-EU: CAPACITOR, European symbol; PARTNO: C067
C4 C21 = rcl:C-EU: CAPACITOR, European symbol; DNP: T; PARTNO: C218; SPICEPREFIX: C
C7 C16 = rcl:CPOL-EU: POLARIZED CAPACITOR, European symbol; PARTNO: C194; SPICEPREFIX: C
C9-C11 C13-C15 C17 C23 C33 C35 C37 C38 C42 C44 C49 C55-C59 = rcl:C-EU: CAPACITOR, European symbol; PARTNO: C216; SPICEPREFIX: C
C12 C18 C19 C24 C30 C47 = rcl:C-EU: CAPACITOR, European symbol; PARTNO: C067; SPICEPREFIX: C
C20 C36 C39 C40 = rcl:C-EU: CAPACITOR, European symbol; PARTNO: C083; SPICEPREFIX: C
C26 C29 = rcl:C-EU: CAPACITOR, European symbol; DNP: T; PARTNO: C020; SPICEPREFIX: C
C31 = rcl:C-EU: CAPACITOR, European symbol; PARTNO: C043; SPICEPREFIX: C
C34 C51 C53 = rcl:C-EU: CAPACITOR, European symbol; PARTNO: C055; SPICEPREFIX: C
C41 C46 = rcl:C-EU: CAPACITOR, European symbol; PARTNO: C028; SPICEPREFIX: C
C43 C45 = resistor:C-EU: CAPACITOR, European symbol; PARTNO: C022
C54 = resistor:C-EU: CAPACITOR, European symbol; PARTNO: C055
D1 = diode:SUPPRESSOR-: Suppressor diode; PARTNO: D087
D2 = diode:SUPPRESSOR-: Suppressor diode; DNP: T; PARTNO: D211
D3 = diode:ZENER-DIODE: Z-Diode; DNP: T; PARTNO: D007
D4 D9 D11-D13 = diode:BAS70: Silicon Schottky Diodes; PARTNO: D204
D5-D7 D10 = diode:SUPPRESSOR-: Suppressor diode; PARTNO: D211
D8 D14 = diode:ZENER-DIODE: Z-Diode; PARTNO: D022
F1 = SSQ250-1K:SSQ250-1K: Square Ceramic Surface Mount Quick Acting Fuse; PARTNO: EM144
F2 F3 = SSQ250-1K:SSQ250-1K: Square Ceramic Surface Mount Quick Acting Fuse; PARTNO: EM186
F4 = SSQ250-1K:SSQ250-1K: Square Ceramic Surface Mount Quick Acting Fuse; PARTNO: EM216
H1 H2 H4 = holes:MOUNT-PAD-ROUND: MOUNTING PAD, round; BOM: EXCLUDE
H3 = holes:MOUNT-HOLE: MOUNTING HOLE with drill center marker; BOM: EXCLUDE; PARTNO: *
IC1 = BTS443:BTS443: Smart Highside Power Switch; PARTNO: IC367
IC2 = texas:ISO1176: ISOLATED RS-485 PROFIBUS TRANSCEIVER Source: Data sheet; MPN: ISO1176DW; OC_FARNELL: 1755037; OC_NEWARK: 13N4111; PARTNO: IC002
IC3 IC4 = MAX15062A:MAX15062A: 60V, 300mA, Ultra-Small, High-Efficiency, Synchronous Step-Down DC-DC Converters; PARTNO: IC292
IC5 IC6 = INA281B:INA281B: INA281-Q1 AEC-Q100, –4-V to 110-V, 1.3-MHz Current-Sense Amplifier; PARTNO: IC350
IC7 IC8 = linear-technology:LT6231: 215MHz, Rail-to-Rail Output, 1.1nV/Hz, 3.5mA Op Amp Source: http://cds.linear.com/docs/Datasheet/623012fb.pdf; MPN: LT6231IS8; OC_FARNELL: unknown; OC_NEWARK: 57M9356; PARTNO: IC222
IC9 = TS912:TS912: Rail-to-rail CMOS dual operational amplifier; PARTNO: IC347
IC10 = TLC555:TLC555: TLC555 LinCMOS™ Timer; PARTNO: IC322
IC11 = STM32G070CB:STM32G070CB: Arm® Cortex®-M0+ 32-bit MCU, 128 KB Flash, 36 KB RAM, 4x USART, timers, ADC, comm. I/Fs, 2.0-3.6V; PARTNO: IC321
IC12 IC13 = LTC6090:LTC6090: 140V CMOS Rail-to-Rail Output, Picoamp Input Current Op Amp; PARTNO: IC330
J1 = Wurth_Connectors_WR-TBL Pluggable Connector:691322110005: WR-TBL Serie 3221 - 3.50 mm Horizontal PCB Header KIND PROPERTIES Pitch 3.5 mm MATERIAL PROPERTIES Insulator Material PA66 Insulator Flammability Rating UL94 V-0 Contact Material Brass Contact Plating Tin GENERAL INFORMATION Operating Temperature -40 up to +105 °C Compliance RoHS ELECTRICAL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; DATASHEET-URL: https://www.we-online.com/catalog/datasheet/691322110005.pdf; IR-UL: 10A; IR-VDE: 10.5A; MOUNT: THT; PART-NUMBER: 691322110005; PARTNO: CON215; PINS: 5; PITCH: 3.5mm; TYPE: Horizontal; VALUE: 691322110005; WORKING-VOLTAGE-UL: 300V (AC); WORKING-VOLTAGE-VDE: 300V (AC)
J2 J3 = Wire-to-Board (rev18a):61200621721: WR-BHD 2.54mm Male Angled Box Header, 6 Pins=>Code : Con_WTB_BHD_2.54_Male_THT_WS_61200621721 Details see: http://katalog.we-online.de/en/em/612_0xx_217_21 Created 2014-06-05, Karrer Zheng 2014 (C) Würth Elektronik; PARTNO: CON398
K1 = Wuerth_Elektronik_eiCan_14_Terminal_Blocks_WR-TBL_2_0:691322110004: WR-TBL Serie 3221 - 3.50mm Horizontal PCB Header, 4 Pins; PARTNO: CON214
K2 = Wuerth_Elektronik_eiCan_14_Terminal_Blocks_WR-TBL_2_0:691322110006: WR-TBL Serie 3221 - 3.50mm Horizontal PCB Header, 6 Pins; PARTNO: CON413
K3 = EB-DIOS M06:EB-DIOSM06: EB-DIOS M06 6-pol. Mini-DIN-Buchse, vollgeschirmt; PARTNO: CON442
K4 = Wuerth_Elektronik_eiCan_09_Wire_to_Board_Connectors (1):61901011021: WR-WTB 2.54mm Right Angled Locking Header Bottom Locking, 10 Pins; PARTNO: CON058
L1-L3 = PowerMagnetics (rev18e):WE-PD_7332_PLASTIC: SMD Shielded Power Inductor; PARTNO: L110; WE-NUMBER: 7447789147/47uH
LED1 = led:LED: LED; PARTNO: D077
LED2 = led:LED: LED; PARTNO: D078
LED3 = led:LED: LED; PARTNO: D079
Q1 = crystal:CRYSTAL: CRYSTAL; OC_FARNELL: unknown; OC_NEWARK: unknown; PARTNO: Q003
R1-R4 R29 R31 R39 R49-R51 R56 R57 R61 R65 R70 R76 R78 R81 = rcl:R-EU_: RESISTOR, European symbol; PARTNO: R245; SPICEPREFIX: R
R5 R6 R73 R77 = rcl:R-EU_: RESISTOR, European symbol; DNP: T; PARTNO: R245; SPICEPREFIX: R
R7 R15 R36 R54 R58 R59 = rcl:R-EU_: RESISTOR, European symbol; PARTNO: R205; SPICEPREFIX: R
R8 R9 R34 R41 R44 R68 R69 = rcl:R-EU_: RESISTOR, European symbol; PARTNO: R173; SPICEPREFIX: R
R10 R18 R28 R38 R53 = rcl:R-EU_: RESISTOR, European symbol; PARTNO: R221; SPICEPREFIX: R
R11 R16 = rcl:R-EU_: RESISTOR, European symbol; DNP: T; PARTNO: R504; SPICEPREFIX: R
R12 = rcl:R-EU_: RESISTOR, European symbol; PARTNO: R247; SPICEPREFIX: R
R13 = rcl:R-EU_: RESISTOR, European symbol; PARTNO: R253; SPICEPREFIX: R
R14 = rcl:R-EU_: RESISTOR, European symbol; PARTNO: R243; SPICEPREFIX: R
R17 = rcl:R-EU_: RESISTOR, European symbol; PARTNO: R157; SPICEPREFIX: R
R19 R20 R23-R25 R27 = rcl:R-EU_: RESISTOR, European symbol; PARTNO: R508; SPICEPREFIX: R
R21 R22 R26 R33 = rcl:R-EU_: RESISTOR, European symbol; PARTNO: R489; SPICEPREFIX: R
R30 R40 = rcl:R-EU_: RESISTOR, European symbol; PARTNO: R254; SPICEPREFIX: R
R32 R45 = resistor:R-EU_: RESISTOR, European symbol; PARTNO: R245
R35 R42 = rcl:R-EU_: RESISTOR, European symbol; PARTNO: R879; SPICEPREFIX: R
R37 R43 = rcl:R-EU_: RESISTOR, European symbol; PARTNO: R875; SPICEPREFIX: R
R46 R47 = rcl:R-EU_: RESISTOR, European symbol; DNP: T; PARTNO: R209; SPICEPREFIX: R
R48 = rcl:R-EU_: RESISTOR, European symbol; PARTNO: R149; SPICEPREFIX: R
R52 = resistor:R-EU_: RESISTOR, European symbol; PARTNO: R209
R55 R62 = rcl:R-EU_: RESISTOR, European symbol; PARTNO: R165; SPICEPREFIX: R
R60 = resistor:R-EU_: RESISTOR, European symbol; PARTNO: R181
R63 R64 R82 = rcl:R-EU_: RESISTOR, European symbol; PARTNO: R504; SPICEPREFIX: R
R66 R67 R71 R72 R74 R75 R79 R80 = rcl:R-EU_: RESISTOR, European symbol; PARTNO: R622; SPICEPREFIX: R
S1 = switch-dil:DA08: DIL/CODE SWITCH; MPN: MCDA08; OC_FARNELL: 9471561; OC_NEWARK: 26M1092; PARTNO: EM214
SW1 SW2 = Wuerth_Elektronik_Switch_Power_Elements:430182095816: WS-TSS-6x6 mm SMD Tact Switch,4 pins; PARTNO: EM015
T1 T2 T4 T5 T9 T10 = transistor:*-NPN-: NPN Transistror BF959 corrected 2008.03.06; PARTNO: T066
T3 T6 = transistor:*-PNP-: PNP Transistror; PARTNO: T073
T7 T8 = transistor:BC847: NPN TRANSISTOR; PARTNO: T165
TP1-TP4 TP6-TP13 = TP_0.6:TP_0.6; BOM: EXCLUDE; PARTNO: *
TP5 = TP_0.6:TP_0.6; BOM: EXCLUDe; PARTNO: *
U1 = MCP1501-40E_SN:MCP1501-40E/SN: High Precision Buffered Voltage Reference; AVAILABILITY: Unavailable; DESCRIPTION: Series Voltage Reference IC ±0.1% 8-SOIC; MF: Microchip; MP: MCP1501-40E/SN; PACKAGE: SOIC-8 Microchip; PARTNO: IC313; PRICE: None
X1 = A_CONN:PF2X5; PARTNO: CON156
